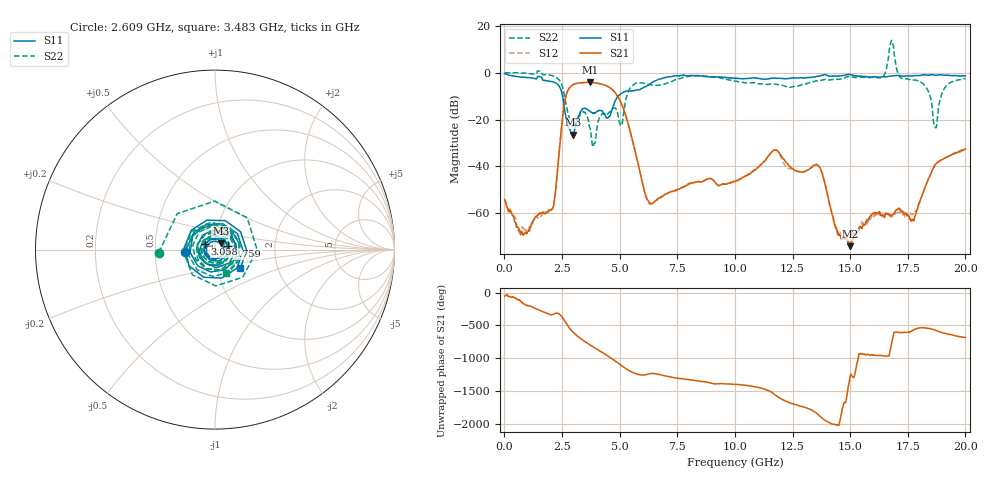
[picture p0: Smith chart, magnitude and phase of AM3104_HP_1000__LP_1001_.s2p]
!Created with skrf (http://scikit-rf.org).
# Hz S RI R 50.0
!freq ReS11 ImS11 ReS21 ImS21 ReS12 ImS12 ReS22 ImS22
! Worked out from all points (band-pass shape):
!   1601 points, 10 MHz to 20 GHz, reference 50 ohm
!   highest |S21| = -4.14 dB at 3.708 GHz (marker M1); lowest = -73.9 dB at 14.99 GHz (marker M2)
!   |S21| within 3 dB of the highest: 2.781 GHz to 4.669 GHz (1.888 GHz wide, 50.7 % of centre)
!   lowest |S11| = -26.5 dB at 2.971 GHz (marker M3), VSWR 1.10, Z = 53.2 + j3.73 ohm
!   |S11| at or under -10 dB: 2.525 GHz to 4.944 GHz (2.419 GHz wide, 64.8 % of centre)
!   |S22| runs from -31.7 to 13.7 dB; largest |S21 - S12| = 0.048
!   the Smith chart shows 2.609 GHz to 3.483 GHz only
!   S11 on the Smith chart (normalised r, x): 2.609 GHz: 0.71, -0.02; 2.759 GHz: 1.15, +0.04; 3.058 GHz: 0.89, +0.06; 3.483 GHz: 1.30, -0.28
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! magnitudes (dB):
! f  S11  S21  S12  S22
! 10 MHz  -0.4  -54.0  -54.3  0.0
! 784.6 MHz  -1.9  -68.4  -65.9  -0.2
! 2.046 GHz  -3.8  -58.3  -58.3  -1.3
! 2.609 GHz  -15.5  -13.2  -13.2  -10.1
! 2.759 GHz  -22.6  -7.6  -7.6  -17.1
! 2.971 GHz  -26.5  -5.2  -5.3  -23.1
! 3.058 GHz  -24.0  -4.9  -4.9  -22.0
! 3.346 GHz  -16.1  -4.3  -4.4  -16.8
! 3.483 GHz  -15.1  -4.2  -4.3  -16.9
! 3.708 GHz  -16.4  -4.1  -4.2  -23.6
! 4.933 GHz  -10.1  -10.5  -10.5  -18.6
! 6.182 GHz  -5.7  -53.6  -54.2  -5.0
! 6.682 GHz  -3.0  -53.6  -53.9  -5.5
! 10.01 GHz  -2.5  -46.5  -46.3  -3.7
! 11.72 GHz  -2.4  -33.0  -33.1  -4.8
! 13.34 GHz  -2.1  -40.3  -40.2  -4.1
! 14.99 GHz  -0.9  -73.9  -69.9  -1.7
! 16.68 GHz  -1.6  -60.5  -61.3  7.3
! 17.73 GHz  -1.4  -62.4  -60.2  -3.2
! 18.69 GHz  -1.1  -39.2  -39.2  -23.3
! 19.11 GHz  -1.2  -36.5  -36.3  -6.4
! 20 GHz  -1.4  -32.6  -32.4  -2.6
